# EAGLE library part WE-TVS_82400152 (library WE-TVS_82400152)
TVS Diode Array WE-TVS, High Speed Series - Low capazity - No leakage current - Low clamping voltage - high ESD voltage protection -- USB 1.0 - 2.0 Flow Thru Design
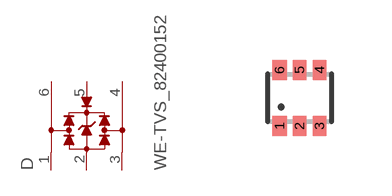
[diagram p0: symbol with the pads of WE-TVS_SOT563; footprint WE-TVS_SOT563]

Designator prefix D

## WE-TVS_82400152 (MPN: 82400152; OC_FARNELL: 1825874; OC_NEWARK: 79R6946; PACKAGE: SOT563; SUPPLIER: Wuerth Elektronik)  [WE-TVS_SOT563]
1  1  pas
2  GND  pwr
3  2  pas
4  3  pas
5  VDD  pwr
6  4  pas

## Footprint WE-TVS_SOT563 (pad centres in mm)
TVS Diode Array WE-TVS
smd 0.35 x 0.5: 1 -0.5,-0.7; 2 0,-0.7; 3 0.5,-0.7; 4 0.5,0.7; 5 0,0.7; 6 -0.5,0.7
